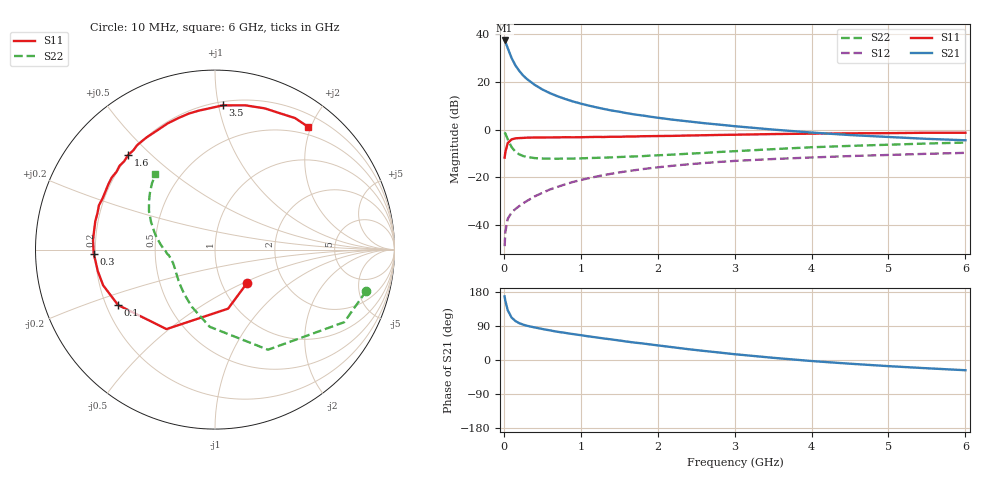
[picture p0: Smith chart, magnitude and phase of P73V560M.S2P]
! SIEMENS Small Signal Semiconductors
! BFP196
! Si NPN RF Bipolar Junction Transistor in SOT143
! VCE = 3.5 V  IC = 60 mA
! Common Emitter S-Parameters:  May  1996
# GHz  S  MA  R  50
!  f  S11  S21  S12  S22
! GHz  MAG  ANG  MAG  ANG  MAG  ANG  MAG  ANG
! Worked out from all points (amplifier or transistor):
!   36 points, 10 MHz to 6 GHz, reference 50 ohm
!   highest |S21| = 37.4 dB at 10 MHz (marker M1)
!   |S21| within 3 dB of that: start of sweep to 48.22 MHz
!   unconditionally stable (mu >= 1): 424.2 MHz to 4.494 GHz
!   at 250 MHz: K = 0.88, MSG = 26.8 dB, |S12| = -30.9 dB
!   at 1.4 GHz: K = 1.08, MAG = 11.5 dB, |S12| = -18.5 dB
!   at 6 GHz: K = 0.98, MSG = 2.6 dB, |S12| = -9.8 dB
!   S11 on the Smith chart (normalised r, x): 10 MHz: 1.32, -0.52; 100 MHz: 0.25, -0.25; 300 MHz: 0.19, -0.02; 1.6 GHz: 0.20, +0.42; 3.5 GHz: 0.23, +1.03; 6 GHz: 0.37, +1.95
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0.01  0.258 -46.2  73.75 167.8  0.0036 79.4  0.8735 -15.3
0.02  0.337 -77.5  68.94 155.7  0.0072 69.7  0.826 -29.3
0.05  0.5189 -121.4  51.3 131.6  0.0134 54.2  0.6313 -62.1
0.1  0.6221 -150.2  31.73 112.2  0.0182 49.7  0.4312 -93.9
0.15  0.6543 -162.3  22.23 102.9  0.0216 51.2  0.3437 -112.1
0.2  0.6639 -169.6  17.03 97.2  0.0249 53.9  0.3025 -124.2
0.25  0.6689 -174.5  13.66 93.3  0.0284 57.0  0.2791 -133.4
0.3  0.6762 -178.0  11.47 90.4  0.0319 58.5  0.2671 -139.4
0.4  0.6816 175.5  8.685 85.9  0.0397 61.9  0.2529 -148.6
0.5  0.6817 171.2  6.94 81.9  0.0471 63.0  0.2471 -154.5
0.6  0.6852 166.8  5.793 78.1  0.0556 63.8  0.2456 -158.6
0.7  0.6858 162.7  4.976 74.4  0.0632 64.0  0.2451 -161.6
0.8  0.6922 159.1  4.363 71.5  0.0714 63.2  0.2467 -164.1
0.9  0.6882 155.5  3.879 68.4  0.0799 62.5  0.2469 -166.3
1.1  0.697 148.4  3.192 62.4  0.0954 60.8  0.2528 -169.4
1.6  0.7153 132.7  2.203 48.6  0.1337 54.3  0.2702 -176.1
2.2  0.7376 116.1  1.609 33.6  0.1748 45.4  0.299 175.9
2.8  0.7718 100.9  1.27 19.7  0.2099 36.5  0.3393 166.7
3.5  0.805 86.8  1 5.8  0.2414 26.4  0.3887 156.5
4.5  0.8343 70.6  0.768 -9.8  0.2784 14.5  0.455 143.9
5.5  0.8577 58.7  0.639 -21.8  0.3104 3.8  0.5098 133.5
6  0.8586 52.9  0.597 -27.0  0.3252 -1.9  0.5344 128.4
